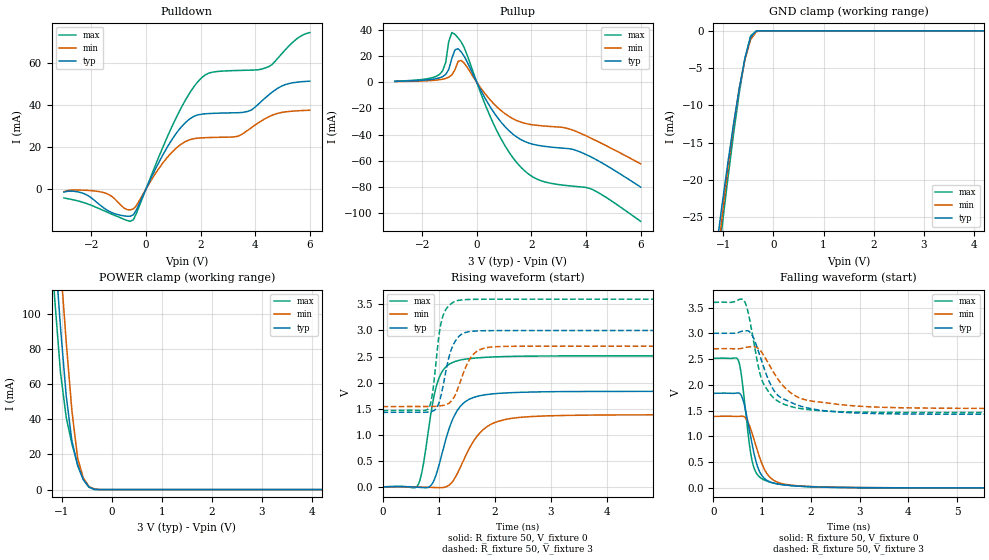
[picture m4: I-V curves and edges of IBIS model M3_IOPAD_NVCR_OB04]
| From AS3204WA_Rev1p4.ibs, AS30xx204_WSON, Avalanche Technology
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[Model] M3_IOPAD_NVCR_OB04
Model_type I/O
Enable   Active-High
Vinl  =  0.9
Vinh  =  2.1
Vmeas =  1.5
Cref  =  30e-12
| Capacitance  typ   min   max
C_comp   3.872127e-12   3.590660e-12   4.176448e-12
| Variables   typ   min   max
[GND Clamp Reference]   0   0   0
[POWER Clamp Reference]   3   2.7   3.6
[Pulldown Reference]   0   0   0
[Pullup Reference]   3   2.7   3.6
[Temperature Range]   25   105   -40
[Voltage Range]   3   2.7   3.6
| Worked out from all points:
|   slope of the pulldown table from 0 to 0.45 V, typ, clamps not added: 37.1 ohm
|   slope of the pullup table from 0 to 0.45 V, typ, clamps not added: 25.9 ohm
|   GND clamp passes 1 mA (typ) near -0.46 V on its own axis
|   POWER clamp passes 1 mA (typ) near -0.42 V on its own axis
|   falling waveform, R_fixture 50, V_fixture 0: 20-80 % time 256ps typ, 321ps min, 201ps max; typ from 1.83 V to 0 V
|   falling waveform, R_fixture 50, V_fixture 3: 20-80 % time 490ps typ, 612ps min, 350ps max; typ from 3 V to 1.43 V
|   rising waveform, R_fixture 50, V_fixture 0: 20-80 % time 339ps typ, 461ps min, 243ps max; typ from 0 V to 1.83 V
|   rising waveform, R_fixture 50, V_fixture 3: 20-80 % time 204ps typ, 266ps min, 147ps max; typ from 1.43 V to 3 V
[GND Clamp]
| Voltage   I(typ)   I(min)   I(max)
-3V       -145.9mA   -151.9mA   -144.2mA
-1.138V   -29.07mA   -31.55mA   -32.68mA
-1.024V   -23.24mA   -24.83mA   -26.15mA
-910.3mV  -17.69mA   -18.46mA   -19.83mA
-796.6mV  -12.47mA   -12.67mA   -13.82mA
-682.8mV  -7.718mA   -7.754mA   -8.316mA
-569mV    -3.663mA   -3.867mA   -3.675mA
-455.2mV  -839.2uA   -1.152mA   -666.1uA
-341.4mV  -35.63uA   -111.1uA   -11.17uA
-113.8mV  -8.642nA   -188.3nA   -1.888nA
6V        0A         0A         0A
[POWER Clamp]
| Voltage   I(typ)   I(min)   I(max)
-3V       949.8mA    984.2mA    923.5mA
-1.252V   183.6mA    221.4mA    154mA
-1.138V   136.7mA    174.2mA    107.6mA
-1.024V   92.09mA    128.1mA    66.35mA
-910.3mV  53.33mA    83.97mA    41.06mA
-796.6mV  27.72mA    44.75mA    25.94mA
-682.8mV  13.75mA    18.06mA    14.29mA
-569mV    5.664mA    6.605mA    5.738mA
-455.2mV  1.446mA    1.789mA    1.305mA
-341.4mV  77.09uA    287.6uA    62.73uA
-227.6mV  1.148uA    12.92uA    332nA
6V        0A         0A         0A
[Pulldown]
| Voltage   I(typ)   I(min)   I(max)
-3V       -1.433mA   -1.188mA   -4.157mA
-2.276V   -2.108mA   -517.7uA   -6.425mA
-1.593V   -8.473mA   -1.507mA   -9.973mA
-455.2mV  -12.21mA   -9.42mA    -14.49mA
931mV     23.15mA    17.28mA    29.13mA
1.448V    31.69mA    22.63mA    42.45mA
1.966V    35.52mA    24.35mA    52.07mA
2.483V    36.1mA     24.62mA    55.8mA
3.745V    37.06mA    28.17mA    56.63mA
4.49V     44.79mA    34.41mA    58.29mA
5.11V     49.81mA    36.8mA     66.46mA
6V        51.42mA    37.57mA    74.56mA
[Pullup]
| Voltage   I(typ)   I(min)   I(max)
-3V       653.5uA    487.7uA    766.8uA
-1.366V   3.311mA    1.902mA    5.899mA
-1.138V   5.906mA    2.886mA    14.98mA
-1.024V   9.73mA     3.87mA     31.24mA
-910.3mV  18.3mA     5.605mA    37.88mA
-796.6mV  24.73mA    9.674mA    36.53mA
-569mV    23.14mA    16.61mA    30.71mA
620.7mV   -22.92mA   -16.38mA   -32.1mA
1.655V    -44.22mA   -30.74mA   -65.72mA
2.379V    -48.66mA   -33.29mA   -75.39mA
3.745V    -52.9mA    -38.5mA    -79.8mA
6V        -80.07mA   -62.32mA   -106.2mA
[Ramp]
dV/dt_r   1.10101/0.339017n  0.831927/0.461224n  1.50845/0.242789n
dV/dt_f   0.94313/0.490001n  0.695697/0.612195n  1.28285/0.349771n
R_load = 50
[Falling Waveform]
R_fixture = 50
V_fixture = 0
V_fixture_min = 0
V_fixture_max = 0
| Time   V(typ)   V(min)   V(max)
0s        1.835V     1.387V     2.514V
508.1ps   1.842V     1.388V     2.484V
563ps     1.81V      1.393V     2.266V
628.4ps   1.639V     1.383V     1.772V
754.2ps   1.042V     1.175V     742mV
850.8ps   600.9mV    886.9mV    345.7mV
956.7ps   299.5mV    569.6mV    204.1mV
1.112ns   137.8mV    259.2mV    126.2mV
1.514ns   51.15mV    62.52mV    51.11mV
21.88ns   622.8nV    711.5nV    10.89uV
[Falling Waveform]
R_fixture = 50
V_fixture = 3
V_fixture_min = 2.7
V_fixture_max = 3.6
| Time   V(typ)   V(min)   V(max)
0s        3V         2.7V       3.6V
624.2ps   3.048V     2.717V     3.642V
788.3ps   2.977V     2.741V     3.046V
963.4ps   2.539V     2.667V     2.19V
1.115ns   2.134V     2.441V     1.888V
1.308ns   1.809V     2.134V     1.693V
1.506ns   1.7V       1.909V     1.603V
2.036ns   1.53V      1.682V     1.509V
4.777ns   1.43V      1.545V     1.463V
21.88ns   1.428V     1.54V      1.462V
[Rising Waveform]
R_fixture = 50
V_fixture = 0
V_fixture_min = 0
V_fixture_max = 0
| Time   V(typ)   V(min)   V(max)
0s        414.5nV    452.2nV    10.8uV
619.8ps   -611.3uV   5.242mV    21.45mV
717.4ps   -8.991mV   2.623mV    378.7mV
871ps     45.71mV    -3.239mV   1.477V
1.013ns   453.4mV    -9.161mV   2.11V
1.262ns   1.331V     129.2mV    2.395V
1.571ns   1.696V     791.7mV    2.465V
2.006ns   1.791V     1.241V     2.495V
2.928ns   1.827V     1.365V     2.512V
21.88ns   1.835V     1.387V     2.514V
[Rising Waveform]
R_fixture = 50
V_fixture = 3
V_fixture_min = 2.7
V_fixture_max = 3.6
| Time   V(typ)   V(min)   V(max)
0s        1.428V     1.54V      1.462V
810.7ps   1.438V     1.544V     1.497V
887.5ps   1.456V     1.544V     1.779V
1.003ns   1.607V     1.552V     2.894V
1.068ns   1.883V     1.562V     3.253V
1.21ns    2.592V     1.633V     3.502V
1.401ns   2.923V     2.069V     3.585V
1.668ns   2.99V      2.593V     3.597V
2.078ns   2.998V     2.692V     3.599V
21.88ns   3V         2.7V       3.6V
